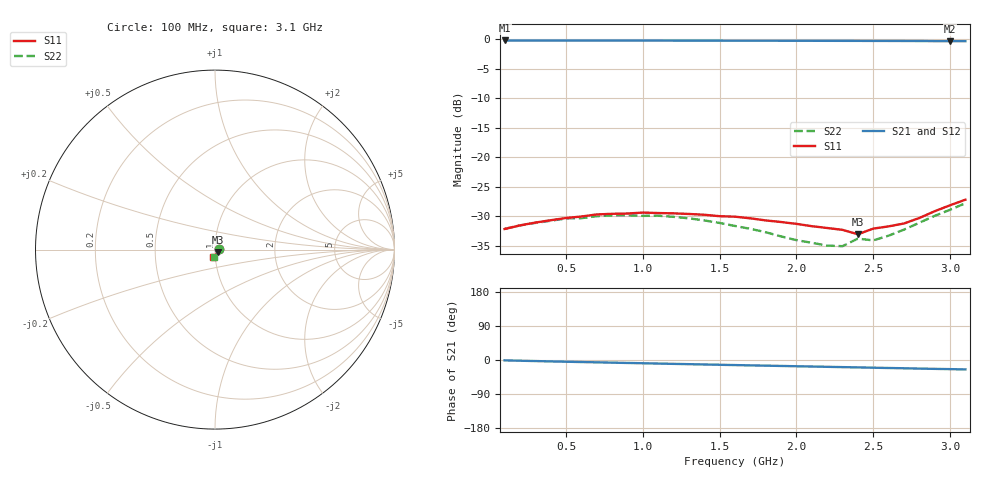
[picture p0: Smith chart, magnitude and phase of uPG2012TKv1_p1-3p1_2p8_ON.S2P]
! NEC Compound Semiconductor Devices Ltd.
! 21.January 2005
! uPG2012TK
! GaAs MMIC (0.1 - 3.1GHz SPDT switch)
! VDD=2.8v Vcont=2.8v / IN-OUT1 ( ON )
! OUT2:50ohm termination
#  GHz  S  MA  R  50
!  f  S11  S21  S12  S22
!  GHz  MAG  ANG  MAG  ANG  MAG  ANG  MAG  ANG
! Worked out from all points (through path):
!   31 points, 100 MHz to 3.1 GHz, reference 50 ohm
!   highest |S21| = -0.21 dB at 100 MHz (marker M1); lowest = -0.3 dB at 3 GHz (marker M2)
!   group delay of S21, straight-line fit = 22 ps
!   lowest |S11| = -33.1 dB at 2.4 GHz (marker M3), VSWR 1.05, Z = 51.6 - j1.55 ohm
!   |S11| at or under -10 dB: start of sweep to end of sweep
!   |S22| runs from -35.1 to -27.8 dB; largest |S21 - S12| = 0.0031
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0.1  0.0246 8.1  0.976 -1.0  0.9761 -1.0  0.0247 8.1
0.3  0.0279 15.7  0.9745 -2.8  0.975 -2.8  0.0277 17.3
0.5  0.0305 19.1  0.9741 -4.5  0.9744 -4.5  0.0302 22.2
0.6  0.0314 21.4  0.9734 -5.4  0.9745 -5.4  0.0304 24.1
0.7  0.0327 20.3  0.9734 -6.1  0.9741 -6.2  0.0316 24.8
0.8  0.0331 19.7  0.9735 -7.0  0.9742 -7.0  0.0321 25.5
1  0.0339 18.6  0.9731 -8.6  0.973 -8.7  0.0318 26.3
1.1  0.0336 16.6  0.9731 -9.4  0.9736 -9.5  0.0319 25.1
1.3  0.033 12.6  0.9724 -11.0  0.9728 -11.0  0.0303 23.0
1.6  0.0313 4.3  0.9713 -13.4  0.9722 -13.4  0.0261 16.1
1.8  0.0291 -4.0  0.971 -14.9  0.9717 -15.0  0.0231 8.3
2  0.0272 -14.5  0.9702 -16.5  0.9708 -16.5  0.0198 -3.5
2.1  0.026 -20.7  0.9696 -17.2  0.9703 -17.3  0.0188 -12.3
2.2  0.0251 -28.6  0.9688 -18.0  0.9701 -18.0  0.0178 -22.1
2.3  0.0242 -37.1  0.9685 -18.8  0.9695 -18.8  0.0176 -33.0
2.4  0.0222 -42.6  0.968 -19.5  0.969 -19.6  0.0204 -44.7
2.5  0.0248 -56.6  0.9673 -20.3  0.968 -20.3  0.0197 -55.5
2.6  0.0259 -68.1  0.967 -21.1  0.9669 -21.1  0.0216 -65.6
2.7  0.0274 -78.0  0.9662 -21.8  0.9659 -21.9  0.0243 -73.7
2.8  0.0305 -86.5  0.965 -22.7  0.9658 -22.6  0.0278 -80.9
3  0.0391 -101.5  0.962 -24.1  0.9646 -24.2  0.0358 -92.1
3.1  0.0436 -106.7  0.9622 -24.9  0.9633 -25.0  0.0407 -96.2
